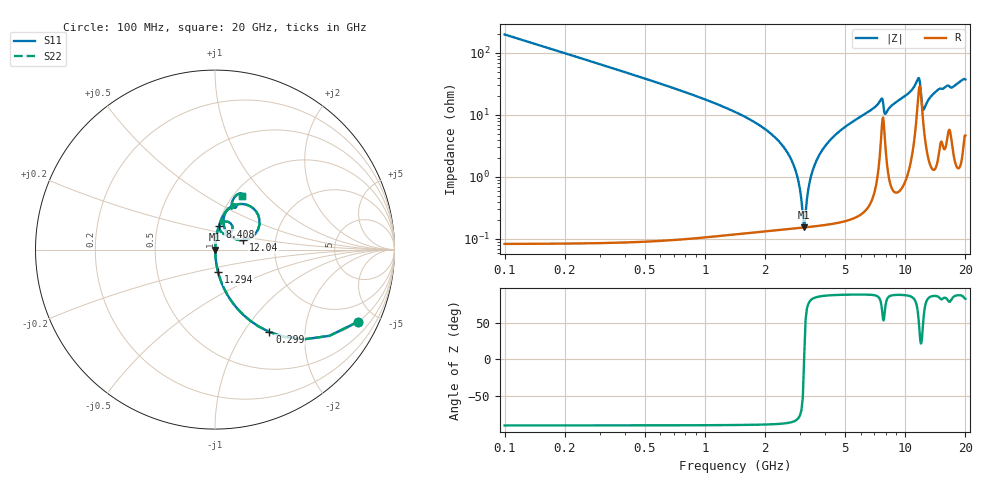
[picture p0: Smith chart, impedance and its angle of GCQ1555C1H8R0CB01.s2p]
!Murata Part Number: GCQ1555C1H8R0CB01
!These Parameters are Measured in Series Mode Connection
!Data Generated on Mar 13, 2026
!  o--ll--o
!Port1  Port2
!  o------o
!Operation Temp=25[degC], DC Bias Voltage=0[V]
!Freq. Start=100[MHz] Stop=20[GHz] 401[Steps]
# Hz S RI R 50
!Freq.(Hz) S11(Real) S11(Imag) S21(Real) S21(Imag) S12(Real) S12(Imag) S22(Real) S22(Imag)
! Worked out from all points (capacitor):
!   401 points, 100 MHz to 20 GHz, reference 50 ohm
!   read as one part in series: C = 8 pF near 199.5 MHz
!   lowest |Z| = 154 mohm at 3.135 GHz (marker M1)
!   series resonance near 3.132 GHz, so ESL is about 320 pH
!   S11 on the Smith chart (normalised r, x): 100 MHz: 1.00, -3.97; 299 MHz: 1.00, -1.32; 1.294 GHz: 1.00, -0.25; 8.408 GHz: 1.02, +0.27; 12.04 GHz: 1.37, +0.15; 20 GHz: 1.09, +0.74
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1e8  0.7979 -0.4014  0.2021 0.4014  0.2021 0.4014  0.7979 -0.4014
2.99e8  0.3032 -0.459  0.6968 0.459  0.6968 0.459  0.3032 -0.459
5.975e8  0.094 -0.2904  0.906 0.2904  0.906 0.2904  0.094 -0.2904
1.294e9  0.0171 -0.1252  0.9829 0.1252  0.9829 0.1252  0.0171 -0.1252
2.5875e9  0.00204 -0.0244  0.998 0.0244  0.998 0.0244  0.00204 -0.0244
2.83625e9  0.00164 -0.0126  0.9984 0.0126  0.9984 0.0126  0.00164 -0.0126
3.03525e9  0.00153 -0.00399  0.9985 0.00399  0.9985 0.00399  0.00153 -0.00399
3.13475e9  0.00153 0.000123  0.9985 -0.000123  0.9985 -0.000123  0.00153 0.000123
3.43325e9  0.00172 0.0118  0.9983 -0.0118  0.9983 -0.0118  0.00172 0.0118
3.83125e9  0.00233 0.0261  0.9977 -0.0261  0.9977 -0.0261  0.00233 0.0261
4.42825e9  0.00386 0.0457  0.9961 -0.0457  0.9961 -0.0457  0.00386 0.0457
6.7665e9  0.0181 0.1179  0.9819 -0.1179  0.9819 -0.1179  0.0181 0.1179
7.61225e9  0.0735 0.1547  0.9265 -0.1547  0.9265 -0.1547  0.0735 0.1547
7.9605e9  0.041 0.0914  0.959 -0.0914  0.959 -0.0914  0.041 0.0914
8.40825e9  0.025 0.1292  0.975 -0.1292  0.975 -0.1292  0.025 0.1292
1.005e10  0.0479 0.1934  0.9521 -0.1934  0.9521 -0.1934  0.0479 0.1934
1.159225e10  0.2142 0.2289  0.7858 -0.2289  0.7858 -0.2289  0.2142 0.2289
1.204e10  0.1585 0.0529  0.8415 -0.0529  0.8415 -0.0529  0.1585 0.0529
1.23385e10  0.0744 0.0847  0.9256 -0.0847  0.9256 -0.0847  0.0744 0.0847
1.338325e10  0.0497 0.1818  0.9503 -0.1818  0.9503 -0.1818  0.0497 0.1818
1.67165e10  0.1148 0.2335  0.8852 -0.2335  0.8852 -0.2335  0.1148 0.2335
2e10  0.1506 0.3003  0.8494 -0.3003  0.8494 -0.3003  0.1506 0.3003
